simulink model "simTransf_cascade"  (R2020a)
settings: Solver=ode15s  StartTime=0.0  StopTime=tsim  FixedStep=0.1  MaxStep=1  RelTol=1e-5
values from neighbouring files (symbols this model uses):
  C = m.c*cp.c/(m.h*cp.h)    [eNTU.m]    (also in runTransf.m = [zeros(1,2*N-1),1]; calcblock.m = Fc*cpc/(Fh*cph); Main.m = [zeros(1,2*N-1),1]; Main_OL.m = [zeros(1,2*N-1),1])
  d_tstep = [500 5000 7000 13000]    [runTransf.m]    (also in Main.m = [1000; 1000;2000]; Main_OL.m = 300; runTestCalcBlk.m = 300; runTransfOL.m)
  dFfeed = 0    [runTransf.m]
  dFh = 0    [runTransf.m]    (also in Main.m = 0;0.2*Fh; runTransfOL.m)
  dm = 0    [runTransf.m]
  dTcin = 0    [runTransf.m]    (also in Main.m = 2; runTransfOL.m)
  dTfeed = 0    [runTransf.m]
  dU = 0    [runTransf.m]    (also in runTransfOL.m)
  dvsp = [5;5];vsp0*0    [runTransf.m]    (also in runTransfOL.m = [0;0];vsp0*0)
  Fc0 = 5    [runTransf.m]    (also in Main.m; Main_OL.m; runTestCalcBlk.m; runTransfOL.m)
  Ffeed0 = (1-R)/R*Fh    (= 27)    [runTransf.m]
  Fh = d(1)    [calcblk.m]    (also in calcv.m; calcv0w.m; runTransf.m = 3; TankWithHEXode.m)
  Kc = 1/kM(i)*tau(i)/(tauCM(i)+theta(i))    [runTransf.m]    (also in Main.m = 1/k*tau/(tauC+theta); runTransfOL.m)
  KI = 1/kS(i)*1/tauCS(i)    [runTransf.m]    (also in Main.m = Kp/tauIv; Main_OL.m = 1; runTransfOL.m)
  m0 = taur*Ffeed0    (= 48600)    [runTransf.m]
  nd = size(d0,2)    [runTransf.m]    (also in Main.m; Main_OL.m; runTestCalcBlk.m; runTransfOL.m)
  np = size(p,2)    [runTransf.m]    (also in runH2Psim.m = length(param); Main.m; Main_OL.m; runTestCalcBlk.m)
  nu = 1    [runTransf.m]    (also in runH2Psim.m = length(u0); Main.m; Main_OL.m; runTestCalcBlk.m)
  nx = size(x0,1)    [runTransf.m]    (also in H2P_Turbine_driven.m = param(end); runTD.m = length(x0); H2P_Boiler_driven.m = param(end); runBD.m = length(x0))
  p = [N, Fc0, rhoc, rhoh, U0, A,cpc,cph]    [runTransf.m]    (also in Main.m = [N, Fc0, rhoc, rhoh,U,A,cpc,cph]; Main_OL.m = [N, Fc0, rhoc, rhoh,U,A,cpc,cph]; runTestCalcBlk.m = [N, Fc0, rhoc, rhoh,U,A,cpc,cph]; NonlinearMap.m = [U;A;Fc(i);Fh;cpc;cph;Tcin;Thin])
  tauI = min(tau(i), 4*(tauCM(i)+theta(i)))    [runTransf.m]    (also in Main.m = min(tau,4*(tauC+theta)); runTransfOL.m)
  Tcin = d(2)    [calcblk.m]    (also in calcv.m; calcv0.m; calcv0w.m; calcvE.m)
  Tfeed0 = Fh/Ffeed0*(Thin-Thend(N)) + Thin    [runTransf.m]
  Thsp = Thsp0    [runTransf.m]    (also in Main.m = Thsp0+dThsp; Main_OL.m = Thsp0+dThsp; runTestCalcBlk.m = Thsp0+dThsp; runTransfOL.m)
  Thsp0 = x0(end);  2.971202611676064e+02    [runTransf.m]    (also in Main.m = Thend(end); Main_OL.m = 297.120261168; runTestCalcBlk.m = Thend(end); runTransfOL.m)
  trf = zeros(3,1)    [runTransf.m]    (also in runTransfOL.m)
  tstep = 10000    [runTransf.m]    (also in Main_OL.m = 100; Main.m = 100; runTransfOL.m = 100)
  U0 = 150    [runTransf.m]    (also in runTransfOL.m)
  vsp0 = [v00; Thin + (Fc0* cpc)/(Fh*cph)*(Tcin-x0(1)); Fc0*(Tcin-x0(1))]    [runTransf.m]    (also in runTransfOL.m)
  x0 = [Tcend(1:N)'; Thend(1:N)']    [runTransf.m]    (also in runTD.m = [TE0;TD0;TSh0;MD0; MSh0;w0;TA0;0;0;0;0;0;0;0;0;0]; runBD.m = [TE0;TD0;TSh0;MD0; MSh0;w0;TA0;0;0;0;0;0;0;0;0;0]; runFP.m = [TE0;TD0;TSh0;MD0; MSh0;w0;TA0;0;0;0;0;0;0;0]; runFPV2.m = [TE0;TD0;TSh0;MD0; MSh0;w0;TA0;0;0;0;0;0;0;0])
undefined symbols (not defined in the file or in its folder): TankWithHEXode

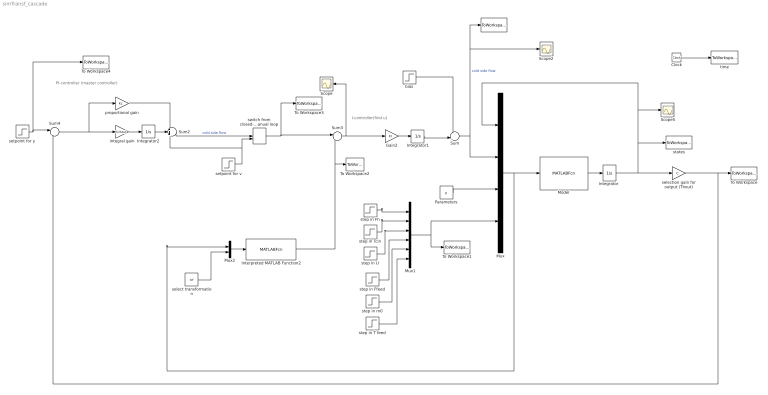
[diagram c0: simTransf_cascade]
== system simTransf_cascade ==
  note: I-controller(find u)
  note: PI-controller (master controller)
  " " : ToWorkspace  VariableName=u  SampleTime=-1
  Clock : Clock
  Gain2 : Gain  Gain=KI  Multiplication=Matrix(K*u)
  "Integrator " : Integrator  InitialCondition=x0
  Integrator1 : Integrator
  Integrator2 : Integrator
  Interpreted MATLAB Function2 : MATLABFcn  MATLABFcn=calcv(u(1:nx),u(nx+1:nx+nu),u(nx+nu+1:nx+nu+np),u(nx+nu+np+1:nx+nu+np+nd),u(end))  OutputDimensions=1
  Model : MATLABFcn  MATLABFcn=TankWithHEXode(u(1:nx),u(nx+1:nx+nu),u(nx+nu+1:nx+nu+np),u(nx+nu+np+1:nx+nu+np+nd))  OutputDimensions=nx  Output1D=off
  Mux : Mux
  Mux1 : Mux  Inputs=6
  Mux2 : Mux  Inputs=2
  Parameters : Constant  Value=p
  Scope : Scope
  Scope2 : Scope
  Scope5 : Scope
  Sum : Sum  Inputs=++|
  Sum2 : Sum  Inputs=+++
  Sum3 : Sum  Inputs=|+-
  Sum4 : Sum  Inputs=|+-
  To Workspace : ToWorkspace  VariableName=Thout  SampleTime=-1
  To Workspace1 : ToWorkspace  VariableName=d  SampleTime=-1
  To Workspace2 : ToWorkspace  VariableName=v  SampleTime=-1
  To Workspace3 : ToWorkspace  VariableName=vs  SampleTime=-1
  To Workspace4 : ToWorkspace  VariableName=ys  SampleTime=-1
  bias : Step  Time=10  Before=Fc0  After=Fc0*1  SampleTime=0
  integral gain : Gain  Gain=Kc/tauI  Multiplication=Matrix(K*u)
  proportional gain : Gain  Gain=Kc  Multiplication=Matrix(K*u)
  select transformation : Constant  Value=trf
  selection gain for output (Thout) : Gain  Gain=C  Multiplication=Matrix(K*u)
  setpoint for v : Step  Time=tstep  Before=vsp0  After=vsp0+dvsp  SampleTime=0
  setpoint for y : Step  Time=tstep  Before=Thsp0  After=Thsp  SampleTime=0
  states : ToWorkspace  VariableName=y  SampleTime=-1
  step in Ffeed : Step  Time=d_tstep(4)  Before=Ffeed0  After=Ffeed0 + dFfeed  SampleTime=0
  step in Fh : Step  Time=d_tstep(1)  Before=Fh  After=Fh+dFh  SampleTime=0
  step in T feed : Step  Time=d_tstep(6)  Before=Tfeed0  After=Tfeed0+dTfeed  SampleTime=0
  step in Tcin : Step  Time=d_tstep(2)  Before=Tcin  After=Tcin+dTcin  SampleTime=0
  step in U : Step  Time=d_tstep(3)  Before=U0  After=U0-dU  SampleTime=0
  step in m0 : Step  Time=d_tstep(5)  Before=m0  After=m0+dm  SampleTime=0
  switch from closed-loop to manual loop : ManualSwitch  CurrentSetting=0
  time : ToWorkspace  VariableName=t  SampleTime=-1
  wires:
  Model/1 -> "Integrator "/1
  "Integrator "/1 -> selection gain for output (Thout)/1, states/1, Mux/1, Scope5/1
  Clock/1 -> time/1
  Parameters/1 -> Mux/3
  Sum/1 -> Mux/2, Scope2/1, " "/1  "cold side flow"
  selection gain for output (Thout)/1 -> Sum4/2, To Workspace/1
  switch from closed-loop to manual loop/1 -> To Workspace3/1, Sum3/1
  Mux1/1 -> Mux/4, To Workspace1/1
  step in Fh/1 -> Mux1/1
  step in Tcin/1 -> Mux1/2
  Gain2/1 -> Integrator1/1
  Sum3/1 -> Gain2/1, Scope/1
  bias/1 -> Sum/1
  Integrator1/1 -> Sum/2
  Mux/1 -> Mux2/1, Model/1
  Interpreted MATLAB Function2/1 -> To Workspace2/1, Sum3/2
  setpoint for v/1 -> switch from closed-loop to manual loop/2, Sum2/3
  Integrator2/1 -> Sum2/2
  integral gain/1 -> Integrator2/1
  proportional gain/1 -> Sum2/1
  Sum2/1 -> switch from closed-loop to manual loop/1  "cold side flow"
  Sum4/1 -> proportional gain/1, integral gain/1
  setpoint for y/1 -> To Workspace4/1, Sum4/1
  step in U/1 -> Mux1/3
  step in Ffeed/1 -> Mux1/4
  step in m0/1 -> Mux1/5
  step in T feed/1 -> Mux1/6
  Mux2/1 -> Interpreted MATLAB Function2/1
  select transformation/1 -> Mux2/2
